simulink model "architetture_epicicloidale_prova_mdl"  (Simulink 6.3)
settings: Solver=ode45  StartTime=0.0  StopTime=3  RelTol=1e-3
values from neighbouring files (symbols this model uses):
  b_c = kb*J_c    (= 4.94590955184)    [architetture_epicicloidale.m]    (also in architetture_epicicloidale_cont.m; architetture_epicicloidale_HEV.m = 92.8974810391; architetture_epicicloidale_prova.m; architetture_HEV_controllo.m = 9.28974810391)
  b_r = kb*J_r    (= 218.026030555)    [architetture_epicicloidale.m]    (also in architetture_epicicloidale_cont.m; architetture_epicicloidale_HEV.m; architetture_epicicloidale_prova.m; architetture_HEV_controllo.m = 21.8026030555)
  b_s = kb*J_s    (= 8.12277148259)    [architetture_epicicloidale.m]    (also in architetture_epicicloidale_cont.m; architetture_epicicloidale_HEV.m = 4.94590955184; architetture_epicicloidale_prova.m; architetture_HEV_controllo.m = 0.494590955184)
  b_sc = kb*J_sc    (= 92.8974810391)    [architetture_epicicloidale.m]    (also in architetture_epicicloidale_cont.m; architetture_epicicloidale_prova.m; epicicloidale.m; epicicloidale_da_solo.m)
  bm = 0.8*N*metri*secondo/rad    (= 0.8)    [architetture_epicicloidale.m]    (also in architetture_epicicloidale_cont.m; architetture_epicicloidale_HEV.m; architetture_epicicloidale_prova.m; architetture_HEV_controllo.m)
  d_cs = d0    (= 10)    [architetture_epicicloidale.m]    (also in architetture_epicicloidale_cont.m; architetture_epicicloidale_prova.m; epicicloidale.m; epicicloidale_da_solo.m)
  d_sr = d0    (= 10)    [architetture_epicicloidale.m]    (also in architetture_epicicloidale_cont.m; architetture_epicicloidale_prova.m; epicicloidale.m; epicicloidale_da_solo.m)
  I_m = eye(m-1)    [architetture_epicicloidale.m]    (also in architetture_epicicloidale_cont.m; architetture_epicicloidale_HEV.m; architetture_epicicloidale_prova.m; architetture_HEV_controllo.m)
  Iw0 = 0*wI0    [architetture_epicicloidale.m]    (also in architetture_epicicloidale_cont.m = wI0; architetture_epicicloidale_HEV.m; architetture_epicicloidale_prova.m; architetture_HEV_controllo.m)
  J_c = 1.3*0.5*pi*rho_acc*hc*r_c^4    (= 0.0494590955184)    [architetture_epicicloidale.m]    (also in architetture_epicicloidale_cont.m; architetture_epicicloidale_HEV.m = 0.928974810391; architetture_epicicloidale_prova.m; architetture_HEV_controllo.m = 0.928974810391)
  J_r = 0.5*pi*rho_acc*(hr*r_ri^4 + h_ring*(r_re^4-r_ri^4))    (= 2.18026030555)    [architetture_epicicloidale.m]    (also in architetture_epicicloidale_cont.m; architetture_epicicloidale_HEV.m; architetture_epicicloidale_prova.m; architetture_HEV_controllo.m)
  J_s = Nr_sat*0.5*pi*rho_acc*(hs*r_s^4 + hc*r_s^4)    (= 0.0812277148259)    [architetture_epicicloidale.m]    (also in architetture_epicicloidale_cont.m; architetture_epicicloidale_HEV.m = 0.0494590955184; architetture_epicicloidale_prova.m; architetture_HEV_controllo.m = 0.0494590955184)
  J_sc = Nr_sat*(r_c+r_s)^2*rho_acc*pi*(hs*r_s^2 + hc*r_s^2)    (= 0.928974810391)    [architetture_epicicloidale.m]    (also in architetture_epicicloidale_cont.m; architetture_epicicloidale_prova.m; epicicloidale.m; epicicloidale_da_solo.m)
  Jm = 1.6*kg*metri^2    (= 1.6)    [architetture_epicicloidale.m]    (also in architetture_epicicloidale_cont.m; architetture_epicicloidale_HEV.m = 1.64945909552; architetture_epicicloidale_prova.m; architetture_HEV_controllo.m = 0.529459095518)
  Jr = Jr([1:m-1],[1:m-1])    [architetture_epicicloidale.m]    (also in architetture_epicicloidale_cont.m; architetture_epicicloidale_HEV.m; architetture_epicicloidale_prova.m; architetture_HEV_controllo.m)
  K_cs = K0    (= 10000000)    [architetture_epicicloidale.m]    (also in architetture_epicicloidale_cont.m; architetture_epicicloidale_prova.m; epicicloidale.m; epicicloidale_da_solo.m)
  K_sr = K0    (= 10000000)    [architetture_epicicloidale.m]    (also in architetture_epicicloidale_cont.m; architetture_epicicloidale_prova.m; epicicloidale.m; epicicloidale_da_solo.m)
  Kf = diag(diag(MLb)'./fliplr(tau_m(1:m-1)))    [architetture_epicicloidale_cont.m]    (also in architetture_epicicloidale_HEV.m; architetture_epicicloidale_prova.m; architetture_HEV_controllo.m; architetture_HEV_startstop.m)
  Kr = Kr([1:m-1])    [architetture_epicicloidale.m]    (also in architetture_epicicloidale_cont.m; architetture_epicicloidale_HEV.m; architetture_epicicloidale_prova.m; architetture_HEV_controllo.m)
  Li = 0.1*Henry    (= 0.1)    [architetture_epicicloidale.m]    (also in architetture_epicicloidale_cont.m; architetture_epicicloidale_HEV.m; architetture_epicicloidale_prova.m; architetture_HEV_controllo.m)
  m = 5    [architetture_epicicloidale.m]    (also in architetture_epicicloidale_cont.m; architetture_epicicloidale_HEV.m; architetture_epicicloidale_prova.m; architetture_HEV_controllo.m)
  Mi = 0.08*Henry    (= 0.08)    [architetture_epicicloidale.m]    (also in architetture_epicicloidale_cont.m; architetture_epicicloidale_HEV.m; architetture_epicicloidale_prova.m; architetture_HEV_controllo.m)
  MKr = MKr([1:m-1],[1:m-1])    [architetture_epicicloidale.m]    (also in architetture_epicicloidale_cont.m; architetture_epicicloidale_HEV.m; architetture_epicicloidale_prova.m; architetture_HEV_controllo.m)
  MLb = MLb([1:m-1],[1:m-1])    [architetture_epicicloidale.m]    (also in architetture_epicicloidale_cont.m; architetture_epicicloidale_HEV.m; architetture_epicicloidale_prova.m; architetture_HEV_controllo.m)
  MR = MR([1:m-1],[1:m-1])    [architetture_epicicloidale.m]    (also in architetture_epicicloidale_cont.m; architetture_epicicloidale_HEV.m; architetture_epicicloidale_prova.m; architetture_HEV_controllo.m)
  Nar = 200    [architetture_epicicloidale.m]    (also in architetture_epicicloidale_cont.m; architetture_epicicloidale_HEV.m; architetture_epicicloidale_prova.m; architetture_HEV_controllo.m)
  Nc = 30    [architetture_epicicloidale.m]    (also in architetture_epicicloidale_cont.m; architetture_epicicloidale_HEV.m; architetture_epicicloidale_prova.m; architetture_HEV_controllo.m)
  Nr_sat = 4    [architetture_epicicloidale.m]    (also in architetture_epicicloidale_cont.m; architetture_epicicloidale_HEV.m; architetture_epicicloidale_prova.m; architetture_HEV_controllo.m)
  p = 1    [architetture_epicicloidale.m]    (also in architetture_epicicloidale_cont.m; architetture_epicicloidale_HEV.m; architetture_epicicloidale_prova.m; architetture_HEV_controllo.m)
  Phir = 0.02*Weber    (= 0.02)    [architetture_epicicloidale.m]    (also in architetture_epicicloidale_cont.m; architetture_epicicloidale_HEV.m; architetture_epicicloidale_prova.m; architetture_HEV_controllo.m)
  r_c = r_ri-2*r_s    (= 0.101859163579)    [architetture_epicicloidale.m]    (also in architetture_epicicloidale_cont.m; architetture_epicicloidale_prova.m; epicicloidale.m; epicicloidale_da_solo.m)
  r_ri = xds*Nr/(2*pi)    (= 0.248281711223)    [architetture_epicicloidale.m]    (also in architetture_epicicloidale_cont.m; architetture_epicicloidale_prova.m; epicicloidale.m; epicicloidale_da_solo.m)
  r_s = xds*Ns/(2*pi)    (= 0.0732112738223)    [architetture_epicicloidale.m]    (also in architetture_epicicloidale_cont.m; architetture_epicicloidale_HEV.m = 0.101859163579; architetture_epicicloidale_prova.m; architetture_HEV_controllo.m = 0.101859163579)
  Ri = 3*Ohm    (= 3)    [architetture_epicicloidale.m]    (also in architetture_epicicloidale_cont.m; architetture_epicicloidale_HEV.m; architetture_epicicloidale_prova.m; architetture_HEV_controllo.m = 0.1)
  Star = Si    [architetture_epicicloidale.m]    (also in architetture_epicicloidale_cont.m; architetture_epicicloidale_HEV.m; architetture_epicicloidale_prova.m; architetture_HEV_controllo.m)
  Tau_sc = 200*N*metri    (= 200)    [architetture_epicicloidale.m]    (also in architetture_epicicloidale_cont.m = 50; architetture_epicicloidale_prova.m = 50; epicicloidale.m = 4; epicicloidale_da_solo.m = 4)
  Tc = 0.05*ms    (= 5e-05)    [architetture_epicicloidale.m]    (also in architetture_epicicloidale_cont.m; architetture_epicicloidale_HEV.m; architetture_epicicloidale_prova.m; architetture_HEV_controllo.m)
  Thm0 = 0    [architetture_epicicloidale.m]    (also in architetture_epicicloidale_cont.m; architetture_epicicloidale_HEV.m; architetture_epicicloidale_prova.m; architetture_HEV_controllo.m)
  tTb = tTb(:,[1:m-1])    [architetture_epicicloidale.m]    (also in architetture_epicicloidale_cont.m; architetture_epicicloidale_HEV.m; architetture_epicicloidale_prova.m; architetture_HEV_controllo.m)
  Wc_0 = 0*0.1*rad/secondo    (= 0)    [architetture_epicicloidale.m]    (also in architetture_epicicloidale_cont.m; architetture_epicicloidale_HEV.m; architetture_epicicloidale_prova.m; Confronto_CVT_EMR.m)
  Wm0 = 0*Wr_d    (= 0)    [architetture_epicicloidale.m]    (also in architetture_epicicloidale_cont.m = 62.5; architetture_epicicloidale_HEV.m; architetture_epicicloidale_prova.m; architetture_HEV_controllo.m)
  Wr_0 = Sys1.C(3,:)*[Wc_0; Wsc_0]    [architetture_epicicloidale.m]    (also in Confronto_CVT_EMR.m = 0; epicicloidale.m; epicicloidale_confronto_statico_elastico.m = [-r_s/r_r, 1+r_s/r_r]*[Ws_0; Wc_0]; epicicloidale_da_solo.m = [ -1/r_ri*r_c, (r_c+r_ri)/r_ri]*[Wc_0; Wsc_0])
  Wsc_0 = -0*0.2*rad/secondo    (= 0)    [architetture_epicicloidale.m]    (also in architetture_epicicloidale_cont.m; architetture_epicicloidale_HEV.m; architetture_epicicloidale_prova.m; epicicloidale.m = -0.2)
undefined symbols (not defined in the file or in its folder): a_0, a_1, B_Pneumatico, DFKc_max, eps_sk, K_Pneumatico, Lambda_mu, Mass_Matrix, Massa_Corpo_Auto, Mu_lambda, Raggio_Ruota_Ant, Raggio_Ruota_Pos, T_omega, tau_a0
libraries: simulink x11, dspmtrx3 x4, Tire_Soil x2, POG_Sincronous_Motors x1

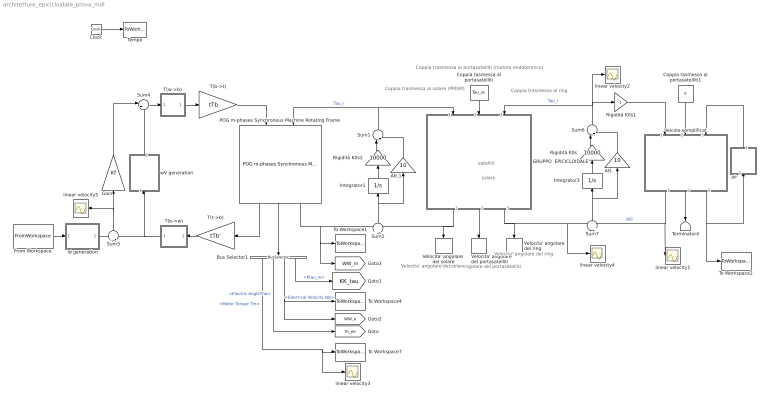
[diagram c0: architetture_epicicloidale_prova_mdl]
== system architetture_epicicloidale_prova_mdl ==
  note: solare
  note: satelliti
  note: Velocita' angolare del portasatelliti
  note: Velocita' angolare del ring
  note: Velocita' angolare del solare
  note: Coppia trasmessa al ring
  note: Coppia trasmessa al solare (PMSM)
  note: Coppia trasmessa ai portasatelliti (motore endotermico)
  " Id generation" : Subsystem
  Att. : Gain  Orientation=up  Gain=10
  Att.1 : Gain  Orientation=up  Gain=10
  Bus Selector1 : BusSelector  Orientation=down  OutputSignals=Motor Torque Tm,Electric AngleThe,Electrical Velocity We,Ktau_w
  Clock : Clock
  Coppia tasmessa al portasatelliti : Constant  Orientation=down  Value=Tau_sc
  Coppia tasmessa al portasatelliti1 : Constant  Orientation=down  Value=0
  From Workspace : FromWorkspace  VariableName=[T_in Tau_des]  SampleTime=0
  GRUPPO  EPICICLOIDALE : Subsystem  Orientation=down  mask(POG Gruppo epicicloidale){Par_solare=[J_c, b_c, r_c], Par_satelliti=[J_s, J_sc, b_s, b_sc, r_s, Nr_sat], Par_ring=[J_r, b_r, r_ri], Tipo_di_Modello=Modello ridotto Wc-Wsc, Cond_in_Wc_Wsc=[Wc_0,  Wsc_0], Cond_in_Wsc_Wr=[Wsc_0,  Wr_0], Cond_in_Wc_Wr=[Wc_0,  Wr_0], Solare_Satelliti=[K_cs, d_cs], Satelliti_Ring=[K_sr, d_sr], Cond_in=[Wc_0, Wsc_0,Wr_0]}
      mask prompts: Par_solare "Parametri Solare: [J_c, b_c, r_c]-->[kg*m^2,N*m*s/rad,m]"; Par_satelliti "Parametri Satelliti: [J_s, J_sc, b_s, b_sc, r_s, Nr_sat]-->[kg*m^2,N*m*s/rad,m]"; Par_ring "Parametri Ring: [J_r, b_r, r_ri]-->[kg*m^2,N*m*s/rad,m,m]"; Tipo_di_Modello "Tipo di modello"; Cond_in_Wc_Wsc "Condizioni iniziali: [Wc_0,  Wsc_0]-->[rad/s]"; Cond_in_Wsc_Wr "Condizioni iniziali: [Wsc_0,  Wr_0]-->[rad/s]"; Cond_in_Wc_Wr "Condizioni iniziali: [Wc_0,  Wr_0]-->[rad/s]"; Solare_Satelliti "Solare-Satelliti: [K_cs, d_cs]-->[N/m,N*m*s/rad]"; Satelliti_Ring "Satelliti-Ring: [K_sr, d_sr]-->[N/m,N*m*s/rad]"; Cond_in "Condizioni iniziali: [Wc_0,  Wsc_0, Wr_0]-->[rad/s]"
      mask help: Gruppo epicicloidale: [J_c, J_s, J_r, J_sc]= Inerzie di: solare, satelliti, ring, solare-ssatelliti; [b_c, b_s, b_r]= Attriti di: solare, satelliti, ring; [r_c, r_s, r_ri, r_re]= Raggi di: solare, satelliti, ring(interno ed esterno); [Nr_sat]= Numero Satelliti; [K_cs, K_sr]= Elasticita' tra solare-satelliti e tra satelliti-ring; [b_sc]= Attriti tra solare-satelliti; [d_cs, d_sr]= Elementi della matrice D; [Wc_0, Wsc_0, Wr_0]=Velocita' iniziali di solare, satelliti, portasatelliti, ring;
      mask init:
      | J_c=double(Par_solare(1));          
      | b_c=double(Par_solare(2));            
      | r_c=double(Par_solare(3));           
      | %
      | J_s=double(Par_satelliti(1));            
      | J_sc=double(Par_satelliti(2));            
      | b_s=double(Par_satelliti(3));            
      | b_sc=double(Par_satelliti(4));            
      | r_s=double(Par_satelliti(5));            
      | Nr_sat=double(Par_satelliti(6));           
      | %
      | J_r=double(Par_ring(1));             
      | b_r=double(Par_ring(2));            
      | r_ri=double(Par_ring(3));                  
      | %
      | %%%%%%%%%%%%%%%%%%%%%%%%%%%%%%%%%%%%%%%%%%%%%%%%%%%%%%%%%%%%%%%%%%%%%%%%%%%
      | %   Modello esteso e modelli ridotti
      | %%%%%%%%%%%%%%%%%%%%%%%%%%%%%%%%%%%%%%%%%%%%%%%%%%%%%%%%%%%%%%%%%%%%%%%%%%%
      | if Tipo_di_Modello=='Modello esteso        '
      |     %
      |     K_cs=double(Solare_Satelliti(1));
      |     d_cs=double(Solare_Satelliti(2));
      |     if(K_cs==0)
      |         K_cs=inf;
      |     end
      |     %
      |     K_sr=double(Satelliti_Ring(1));
      |     d_sr=double(Satelliti_Ring(2));
      |     if(K_sr==0)
      |         K_sr=inf;
      |     end
      |     %
      |     %
      |     L=[ J_c,      0,      0,      0,      0,      0;
      |           0, 1/K_cs,      0,      0,      0,      0;
      |           0,      0,    J_s,      0,      0,      0;
      |           0,      0,      0,   J_sc,      0,      0;
      |           0,      0,      0,      0, 1/K_sr,      0;
      |           0,      0,      0,      0,      0,    J_r];
      |     %
      |     A=- [-b_c-r_c^2*d_cs,    -r_c,                -r_c*d_cs*r_s,                   r_c^2*d_cs,      0,                  0;
      |         r_c,                    0,                          r_s,                         -r_c,      0,                  0;
      |         -r_c*d_cs*r_s,       -r_s,   -b_s-d_cs*r_s^2-d_sr*r_s^2,   r_c*d_cs*r_s-d_sr*r_s*r_ri,   -r_s,      d_sr*r_s*r_ri;
      |         r_c^2*d_cs,           r_c,   r_c*d_cs*r_s-d_sr*r_s*r_ri, -b_sc-r_c^2*d_cs-d_sr*r_ri^2,  -r_ri,        d_sr*r_ri^2;
      |         0,                      0,                          r_s,                         r_ri,      0,              -r_ri;
      |         0,                      0,                d_sr*r_s*r_ri,                  d_sr*r_ri^2,   r_ri,   -b_r-d_sr*r_ri^2];
      |     %
      |     B=[ 1, 0, 0;
      |         0, 0, 0;
      |         0, 0, 0;
      |         0, 1, 0;
      |         0, 0, 0;
      |         0, 0, 1];
      |     %
      |     C=[ 1, 0, 0, 0, 0, 0;
      |         0, 0, 0, 1, 0, 0;
      |         0, 0, 0, 0, 0, 1];
      |     %
      |     Wc_0=double(Cond_in(1));
      |     Wsc_0=double(Cond_in(2));
      |     Wr_0=double(Cond_in(3));
      |     Ws_0=r_c*(Wsc_0-Wc_0)/r_s;
      |     Ws_sc_0=[Ws_0 Wsc_0];
      |     %
      |     We_0=[Wc_0 0 Ws_sc_0 0 Wr_0 ];
      |     %
      | elseif Tipo_di_Modello=='Modello ridotto Wc-Wsc'
      |     L = [ (J_c*r_s^2*r_ri^2+r_ri^2*r_c^2*J_s+J_r*r_s^2*r_c^2)/r_s^2/r_ri^2,                                        -r_c*(r_ri^2*r_c*J_s+J_r*r_s^2*r_c+J_r*r_s^2*r_ri)/r_s^2/r_ri^2;
      |           -r_c*(r_ri^2*r_c*J_s+J_r*r_s^2*r_c+J_r*r_s^2*r_ri)/r_s^2/r_ri^2, (J_r*r_s^2*r_c^2+2*J_r*r_s^2*r_ri*r_c+J_r*r_s^2*r_ri^2+r_ri^2*r_c^2*J_s+r_ri^2*J_sc*r_s^2)/r_s^2/r_ri^2];
      |     %
      |     A=-[ -(b_c*r_s^2*r_ri^2+r_c^2*r_ri^2*b_s+b_r*r_s^2*r_c^2)/r_s^2/r_ri^2,                                          r_c*(r_c*r_ri^2*b_s+b_r*r_s^2*r_c+b_r*r_s^2*r_ri)/r_s^2/r_ri^2;
      |         r_c*(r_c*r_ri^2*b_s+b_r*r_s^2*r_c+b_r*r_s^2*r_ri)/r_s^2/r_ri^2,    -(b_sc*r_s^2*r_ri^2+r_c^2*r_ri^2*b_s+b_r*r_s^2*r_c^2+2*b_r*r_s^2*r_c*r_ri+b_r*r_s^2*r_ri^2)/r_s^2/r_ri^2];
      |     %
      |     B= [  1,    0,     -1/r_ri*r_c;
      |           0,    1, (r_c+r_ri)/r_ri];
      |     %
      |     C= [            1,               0;
      |                     0,               1;
      |           -1/r_ri*r_c, (r_c+r_ri)/r_ri];
      |     %
      |     Wc_0=double(Cond_in_Wc_Wsc(1));
      |     Wsc_0=double(Cond_in_Wc_Wsc(2));
      |     We_0=[Wc_0 Wsc_0];
      |     %
      | elseif Tipo_di_Modello=='Modello ridotto Wsc-Wr'
      |     L= [ (J_sc*r_c^2*r_s^2+J_c*r_s^2*r_c^2+2*J_c*r_s^2*r_c*r_ri+J_c*r_s^2*r_ri^2+r_ri^2*J_s*r_c^2)/r_c^2/r_s^2,   -r_ri*(J_c*r_s^2*r_c+J_c*r_s^2*r_ri+r_ri*J_s*r_c^2)/r_c^2/r_s^2;
      |          -r_ri*(J_c*r_s^2*r_c+J_c*r_s^2*r_ri+r_ri*J_s*r_c^2)/r_c^2/r_s^2,                                        (J_r*r_c^2*r_s^2+J_c*r_s^2*r_ri^2+r_ri^2*J_s*r_c^2)/r_c^2/r_s^2];
      | 
      |     A=-[ -(b_sc*r_c^2*r_s^2+b_c*r_s^2*r_c^2+2*b_c*r_s^2*r_c*r_ri+b_c*r_s^2*r_ri^2+r_ri^2*b_s*r_c^2)/r_c^2/r_s^2,     r_ri*(b_c*r_s^2*r_c+b_c*r_s^2*r_ri+r_ri*b_s*r_c^2)/r_c^2/r_s^2;
      |          r_ri*(b_c*r_s^2*r_c+b_c*r_s^2*r_ri+r_ri*b_s*r_c^2)/r_c^2/r_s^2,                                          -(b_r*r_c^2*r_s^2+b_c*r_s^2*r_ri^2+r_ri^2*b_s*r_c^2)/r_c^2/r_s^2];
      | 
      |     B= [ (r_c+r_ri)/r_c,    1,   0;
      |             -1/r_c*r_ri,    0,   1];
      | 
      |     C= [ (r_c+r_ri)/r_c,  -1/r_c*r_ri;
      |                       1,            0;
      |                       0,            1];
      |     %
      |     Wsc_0=double(Cond_in_Wsc_Wr(1));
      |     Wr_0=double(Cond_in_Wsc_Wr(2));
      |     We_0=[Wsc_0 Wr_0];
      |     %
      | elseif Tipo_di_Modello=='Modello ridotto  Wc-Wr'
      |     L= [ (J_c*r_s^2*r_c^2+2*J_c*r_s^2*r_c*r_ri+J_c*r_s^2*r_ri^2+r_ri^2*r_c^2*J_s+r_c^2*J_sc*r_s^2)/r_s^2/(r_c+r_ri)^2,                                                        r_c*r_ri*(-r_ri*r_c*J_s+J_sc*r_s^2)/r_s^2/(r_c+r_ri)^2;
      |           r_c*r_ri*(-r_ri*r_c*J_s+J_sc*r_s^2)/r_s^2/(r_c+r_ri)^2,                                                      (J_r*r_s^2*r_c^2+2*J_r*r_s^2*r_c*r_ri+J_r*r_s^2*r_ri^2+r_ri^2*r_c^2*J_s+r_ri^2*J_sc*r_s^2)/r_s^2/(r_c+r_ri)^2];
      | 
      |     A=-[-(b_c*r_s^2*r_c^2+2*b_c*r_s^2*r_c*r_ri+b_c*r_s^2*r_ri^2+r_c^2*r_ri^2*b_s+r_c^2*r_s^2*b_sc)/r_s^2/(r_c+r_ri)^2,                                                        -r_c*r_ri*(-r_c*r_ri*b_s+r_s^2*b_sc)/r_s^2/(r_c+r_ri)^2;
      |         -r_c*r_ri*(-r_c*r_ri*b_s+r_s^2*b_sc)/r_s^2/(r_c+r_ri)^2,                                                       -(b_r*r_s^2*r_c^2+2*b_r*r_s^2*r_c*r_ri+b_r*r_s^2*r_ri^2+r_c^2*r_ri^2*b_s+r_ri^2*r_s^2*b_sc)/r_s^2/(r_c+r_ri)^2];
      | 
      |     B=[   1,  1/(r_c+r_ri)*r_c, 0;
      |           0, 1/(r_c+r_ri)*r_ri, 1];
      | 
      |     C=[                 1,                  0;
      |          1/(r_c+r_ri)*r_c,  1/(r_c+r_ri)*r_ri;
      |                         0,                  1];
      |     Wc_0=double(Cond_in_Wc_Wr(1));
      |     Wr_0=double(Cond_in_Wc_Wr(2));
      |     We_0=[Wc_0 Wr_0];
      | end
  Gain : Gain  Orientation=up  Gain=Kf  Multiplication=Matrix(K*u) (u vector)
  Integrator1 : Integrator  Orientation=up
  Integrator3 : Integrator  Orientation=up
  POG m-phases Synchronous Machine Rotating Frame : POG_Sincronous_Motors/POG m-phases Synchronous Machine Rotating Frame  Orientation=down  Motor_Par=[m p]  Phase_Par=[Nc Star]  Electric_Par=[Ri Li Mi]  Mech_Par=[Jm bm]  Plux_Par=[Phir Nar]  Iniz_Cond=[Wm0; Thm0; Iw0]  TipoFlux=User defined  Tipo=Tipo  alfa=al  degree=6  TipoF=Tipo
  Rigidità K0s : Gain  Orientation=up  Gain=10000
  Rigidità K0s1 : Gain  Gain=-1
  Rigidità K0s2 : Gain  Orientation=up  Gain=10000
  Sum1 : Sum  Orientation=up  Inputs=|++
  Sum2 : Sum  Orientation=up  Inputs=+|-
  Sum3 : Sum  Orientation=up  Inputs=+|-
  Sum4 : Sum  Inputs=|++
  Sum6 : Sum  Orientation=up  Inputs=|++
  Sum7 : Sum  Orientation=up  Inputs=-|+
  T(b->t) : Gain  Gain=tTb  Multiplication=Matrix(K*u) (u vector)
  T(b->w) : Subsystem  Orientation=left  AncestorBlock=|
      | POG_Electric_Bloks/POG m-phases
      | Synchronous Machine
      | Rotating Frame/T(b->w)
  T(t->b) : Gain  Orientation=left  Gain=tTb'  Multiplication=Matrix(K*u) (u vector)
  T(w->b) : Subsystem  AncestorBlock=|
      | POG_Electric_Bloks/POG m-phases
      | Synchronous Machine
      | Rotating Frame/T(w->b)
  Tempo : ToWorkspace  VariableName=t  SampleTime=Tc  SaveFormat=Array
  Terminator4 : Terminator
  To Workspace1 : ToWorkspace  VariableName=Wm  SampleTime=Tc  SaveFormat=Array
  To Workspace2 : ToWorkspace  VariableName=Vvehicle  SampleTime=Tc  SaveFormat=Array
  To Workspace4 : ToWorkspace  VariableName=We  SampleTime=Tc  SaveFormat=Array
  To Workspace7 : ToWorkspace  VariableName=Tm  SampleTime=Tc  SaveFormat=Array
  Veicolo semplificat : Subsystem  Orientation=down
  Velocita' angolare del ring : ToWorkspace  VariableName=W_r  SampleTime=Tc  SaveFormat=Array
  Velocita' angolare  del portasatelliti : ToWorkspace  VariableName=W_sc  SampleTime=Tc  SaveFormat=Array
  Velocita' angolare  del solare : ToWorkspace  VariableName=W_c  SampleTime=Tc  SaveFormat=Array
  air : Subsystem  Orientation=up
  linear velocity{1..5} (5 alike) : Scope
  wV generation : Subsystem  Orientation=up
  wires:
  Clock/1 -> Tempo/1
  Coppia tasmessa al portasatelliti/1 -> GRUPPO  EPICICLOIDALE/2(Tau_sc)
  GRUPPO  EPICICLOIDALE/3(w_r) -> Velocita' angolare del ring/1, Sum7/1, linear velocity4/1
  GRUPPO  EPICICLOIDALE/2(w_sc) -> Velocita' angolare  del portasatelliti/1
  GRUPPO  EPICICLOIDALE/1(w_c) -> Velocita' angolare  del solare/1, Sum2/2
  POG m-phases Synchronous Machine Rotating Frame/3 -> Sum2/1, To Workspace1/1, [WW_m]
  POG m-phases Synchronous Machine Rotating Frame/2 -> Bus Selector1/1
  Bus Selector1/3 -> To Workspace4/1, [WW_e]  "<Electrical Velocity We>"
  T(w->b)/1(It) -> T(b->t)/1
  T(b->t)/1 -> POG m-phases Synchronous Machine Rotating Frame/1
  T(t->b)/1 -> T(b->w)/1(Vt)
  T(b->w)/1(Vw) -> wV generation/1(In1), Sum3/2
  POG m-phases Synchronous Machine Rotating Frame/1 -> T(t->b)/1
  Bus Selector1/2 -> [th_ee]  "<Electric AngleThe>"
  Bus Selector1/1 -> To Workspace7/1, linear velocity3/1  "<Motor Torque Tm>"
  Att./1 -> Sum6/2
  Rigidità K0s/1 -> Sum6/1
  Integrator3/1 -> Rigidità K0s/1
  Sum6/1 -> linear velocity2/1, Rigidità K0s1/1, GRUPPO  EPICICLOIDALE/3(Tau_r)  "Tau_r"
  Sum7/1 -> Att./1, Integrator3/1
  Coppia tasmessa al portasatelliti1/1 -> Veicolo semplificat/2(Tau2)
  Rigidità K0s1/1 -> Veicolo semplificat/1(Tau1)
  Att.1/1 -> Sum1/2
  Rigidità K0s2/1 -> Sum1/1
  Integrator1/1 -> Rigidità K0s2/1
  Sum2/1 -> Att.1/1, Integrator1/1
  Sum1/1 -> POG m-phases Synchronous Machine Rotating Frame/2, GRUPPO  EPICICLOIDALE/1(Tau_c)  "Tau_r"
  " Id generation"/1(Out1) -> Sum3/1
  Sum3/1 -> Gain/1, linear velocity5/1
  Sum4/1 -> T(w->b)/1(Iw)
  From Workspace/1 -> " Id generation"/1(In1)
  Gain/1 -> Sum4/1
  wV generation/1(Out1) -> Sum4/2
  Veicolo semplificat/1(W1) -> Sum7/2, linear velocity1/1  "W0"
  Veicolo semplificat/3(V) -> To Workspace2/1, air/1(In1)
  Bus Selector1/4 -> [KK_tau]  "<Ktau_w>"
  air/1(Out1) -> Veicolo semplificat/3(Fres)
  Veicolo semplificat/2(W2) -> Terminator4/1

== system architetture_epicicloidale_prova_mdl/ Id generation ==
  In1 : Inport
  Divide : Product  Inputs=*/  OutScaling=2^-10
  Product : Product
  modulo : Subsystem
  versore : Subsystem
  Out1 : Outport
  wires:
  [KK_tau] -> modulo/1(In1), versore/1(In1)
  modulo/1(Out1) -> Divide/2
  Divide/1 -> Product/1
  versore/1(Out1) -> Product/2
  In1/1 -> Divide/1
  Product/1 -> Out1/1

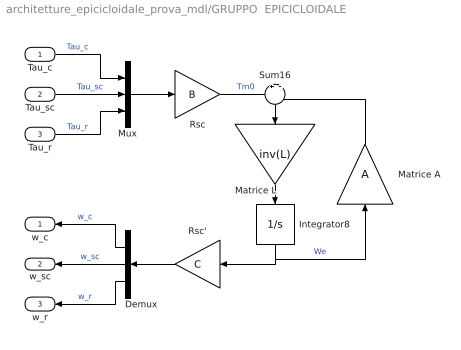
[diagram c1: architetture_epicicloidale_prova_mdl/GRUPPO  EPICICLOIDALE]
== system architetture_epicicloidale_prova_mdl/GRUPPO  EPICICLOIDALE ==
  Tau_c : Inport
  Tau_sc : Inport  Port=2
  Tau_r : Inport  Port=3
  Demux : Demux  Orientation=left  Outputs=3
  Integrator8 : Integrator  Orientation=down  InitialCondition=We_0  LowerSaturationLimit=0
  Matrice A : Gain  Orientation=up  Gain=A  Multiplication=Matrix(K*u)
  Matrice L : Gain  Orientation=down  Gain=inv(L)  Multiplication=Matrix(K*u)
  Mux : Mux  Inputs=3
  Rsc : Gain  Gain=B  Multiplication=Matrix(K*u)
  Rsc' : Gain  Orientation=left  Gain=C  Multiplication=Matrix(K*u)
  Sum16 : Sum  Orientation=down  Inputs=+|-
  w_c : Outport  Orientation=left
  w_sc : Outport  Orientation=left  Port=2
  w_r : Outport  Orientation=left  Port=3
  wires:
  Rsc/1 -> Sum16/1  "Tm0"
  Sum16/1 -> Matrice L/1
  Matrice L/1 -> Integrator8/1
  Integrator8/1 -> Matrice A/1, Rsc'/1  "We"
  Matrice A/1 -> Sum16/2
  Tau_c/1 -> Mux/1  "Tau_c"
  Tau_sc/1 -> Mux/2  "Tau_sc"
  Tau_r/1 -> Mux/3  "Tau_r"
  Mux/1 -> Rsc/1
  Rsc'/1 -> Demux/1
  Demux/1 -> w_c/1  "w_c"
  Demux/2 -> w_sc/1  "w_sc"
  Demux/3 -> w_r/1  "w_r"

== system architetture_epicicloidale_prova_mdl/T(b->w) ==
  Vt : Inport
  Product : Product  Multiplication=Matrix(*)
  Vw : Outport
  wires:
  Vt/1 -> Product/2
  Product/1 -> Vw/1
  [T_w_be] -> Product/1

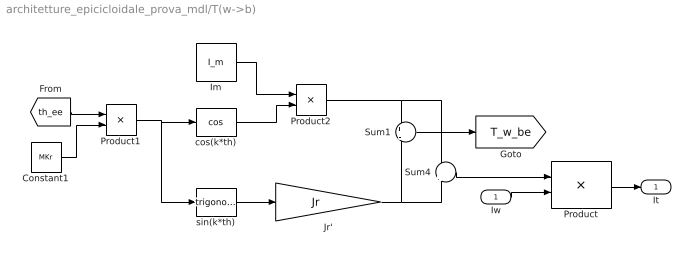
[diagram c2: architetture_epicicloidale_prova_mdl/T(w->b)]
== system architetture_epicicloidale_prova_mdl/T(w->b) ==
  Iw : Inport
  Constant1 : Constant  Value=MKr
  Im : Constant  Value=I_m  VectorParams1D=off
  Jr' : Gain  Gain=Jr  Multiplication=Matrix(K*u)
  Product : Product  Multiplication=Matrix(*)
  Product1 : Product
  Product2 : Product
  Sum1 : Sum  Inputs=+|-
  Sum4 : Sum  Inputs=+|+
  cos(k*th) : Trigonometry  Operator=cos
  sin(k*th) : Trigonometry
  It : Outport
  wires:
  Sum4/1 -> Product/1
  Product/1 -> It/1
  Iw/1 -> Product/2
  Jr'/1 -> Sum4/2, Sum1/2
  Product2/1 -> Sum4/1, Sum1/1
  Im/1 -> Product2/1
  cos(k*th)/1 -> Product2/2
  Product1/1 -> sin(k*th)/1, cos(k*th)/1
  Constant1/1 -> Product1/2
  [th_ee] -> Product1/1
  sin(k*th)/1 -> Jr'/1
  Sum1/1 -> [T_w_be]

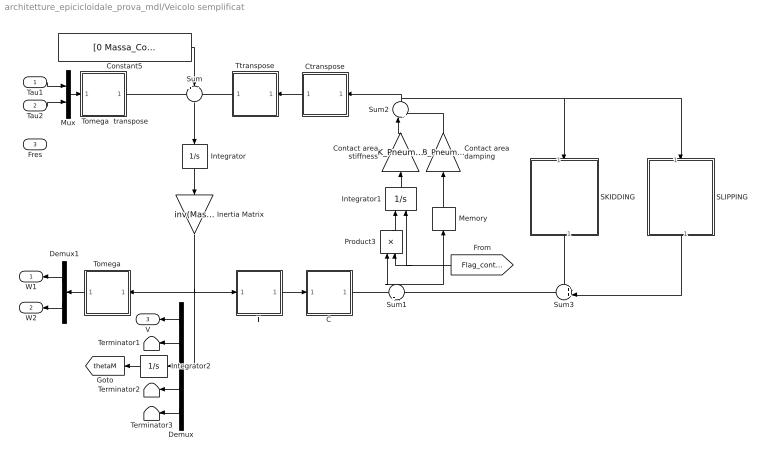
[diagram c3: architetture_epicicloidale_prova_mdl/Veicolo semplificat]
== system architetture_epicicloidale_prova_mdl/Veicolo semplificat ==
  Tau1 : Inport
  Tau2 : Inport  Port=2
  Fres : Inport  Port=3
  C : Subsystem
  Constant5 : Constant  Value=[0 Massa_Corpo_Auto*9.81 0 0 0]
  Contact area damping : Gain  Orientation=up  Gain=B_Pneumatico  Multiplication=Matrix(K*u) (u vector)
  Contact area stiffness : Gain  Orientation=up  Gain=K_Pneumatico  Multiplication=Matrix(K*u) (u vector)
  Ctranspose : Subsystem  Orientation=left
  Demux : Demux  Orientation=left  Outputs=5
  Demux1 : Demux  Orientation=left  Outputs=2
  Inertia Matrix : Gain  Orientation=down  Gain=inv(Mass_Matrix)  Multiplication=Matrix(K*u)
  Integrator : Integrator  Orientation=down  InitialCondition=[0 0 0 0 0]
  Integrator1 : Integrator  Orientation=up  ExternalReset=falling  InitialCondition=[0 0 0 0 0 0]
  Integrator2 : Integrator  Orientation=left
  Memory : Memory  Orientation=up
  Mux : Mux  Inputs=2
  Product3 : Product  Orientation=up  Inputs=**
  SKIDDING : Subsystem  Orientation=down  AncestorBlock=Tire_Soil/Tire-soil contact ENERGETIC/Contatto elastico/SKIDDING
  SLIPPING : Subsystem  Orientation=down  AncestorBlock=Tire_Soil/Tire-soil contact ENERGETIC/Contatto elastico/SLIPPING
  Sum : Sum  Orientation=down  Inputs=+--
  Sum1 : Sum  Orientation=up  Inputs=+-
  Sum2 : Sum  Orientation=up  Inputs=|++
  Sum3 : Sum  Orientation=left  Inputs=++|
  T : Subsystem
  Terminator1 : Terminator
  Terminator2 : Terminator
  Terminator3 : Terminator
  Tomega : Subsystem  Orientation=left
  Tomega  transpose : Subsystem
  Ttranspose : Subsystem  Orientation=left
  W1 : Outport  Orientation=left
  W2 : Outport  Orientation=left  Port=2
  V : Outport  Orientation=left  Port=3
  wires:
  Demux/5 -> Terminator3/1
  Demux/4 -> Terminator2/1
  Demux/2 -> Terminator1/1
  Demux/1 -> V/1
  Tomega/1(Vt) -> Demux1/1
  Tau2/1 -> Mux/2
  Tau1/1 -> Mux/1
  Mux/1 -> Tomega  transpose/1(T)
  Tomega  transpose/1(Tt) -> Sum/1
  Constant5/1 -> Sum/2
  Sum3/1 -> Sum1/2
  SKIDDING/1(Vcsk) -> Sum3/1
  SLIPPING/1(Vcsl) -> Sum3/2
  Memory/1 -> Contact area damping/1
  Integrator1/1 -> Contact area stiffness/1
  Product3/1 -> Integrator1/1
  [Flag_contatto] -> Integrator1/2, Product3/2
  C/1(Xcdot) -> Sum1/1
  Ctranspose/1(F) -> Ttranspose/1(F)
  T/1(Xdot) -> C/1(Xdot)
  Integrator2/1 -> [thetaM]
  Demux/3 -> Integrator2/1
  Contact area stiffness/1 -> Sum2/1
  Contact area damping/1 -> Sum2/2
  Sum1/1 -> Memory/1, Product3/1
  Sum2/1 -> Ctranspose/1(Fc), SLIPPING/1(Fxyz), SKIDDING/1(Fxyz)
  Ttranspose/1(Ft) -> Sum/3
  Inertia Matrix/1 -> T/1(V), Tomega/1(V), Demux/1
  Integrator/1 -> Inertia Matrix/1
  Sum/1 -> Integrator/1
  Demux1/1 -> W1/1
  Demux1/2 -> W2/1

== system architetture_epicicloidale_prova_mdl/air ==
  In1 : Inport  Orientation=up
  air : Fcn  Orientation=up  Expr=10*u^2
  Out1 : Outport  Orientation=up
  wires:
  In1/1 -> air/1
  air/1 -> Out1/1

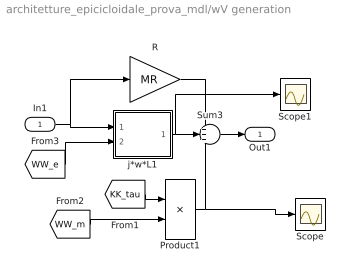
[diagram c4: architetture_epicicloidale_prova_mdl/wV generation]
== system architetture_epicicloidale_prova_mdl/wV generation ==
  In1 : Inport
  Product1 : Product  Multiplication=Matrix(*)
  R : Gain  Gain=MR  Multiplication=Matrix(K*u) (u vector)
  Scope : Scope
  Scope1 : Scope
  Sum3 : Sum  Inputs=+++
  j*w*L1 : Subsystem  AncestorBlock=|
      | POG_Electric_Bloks/POG m-phases
      | Synchronous Machine
      | Rotating Frame/j*w*L
  Out1 : Outport
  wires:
  [KK_tau] -> Product1/1
  [WW_m] -> Product1/2
  R/1 -> Sum3/1
  j*w*L1/1(Out1) -> Sum3/2, Scope1/1
  Product1/1 -> Sum3/3, Scope/1
  In1/1 -> j*w*L1/1(In1), R/1
  Sum3/1 -> Out1/1
  [WW_e] -> j*w*L1/2(In2)

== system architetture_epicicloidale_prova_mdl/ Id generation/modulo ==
  In1 : Inport
  Dot Product : simulink/Math Operations/Dot Product  InputSameDT=on  OutDataType=sfix(16)  OutScaling=2^-10  DoSatur=off
  Math Function : Math  Operator=sqrt
  Out1 : Outport
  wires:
  In1/1 -> Dot Product/1, Dot Product/2
  Dot Product/1 -> Math Function/1
  Math Function/1 -> Out1/1

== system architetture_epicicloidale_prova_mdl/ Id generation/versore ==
  In1 : Inport
  Constant : Constant  Value=0.0001
  Divide : Product  Inputs=*/  OutScaling=2^-10
  Norma  del vettore : Subsystem
  Sum1 : Sum  Inputs=|++
  Out1 : Outport
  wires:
  Divide/1 -> Out1/1  "versore"
  Constant/1 -> Sum1/2
  Sum1/1 -> Divide/2
  Norma  del vettore/1(Out1) -> Sum1/1
  In1/1 -> Norma  del vettore/1(In1), Divide/1

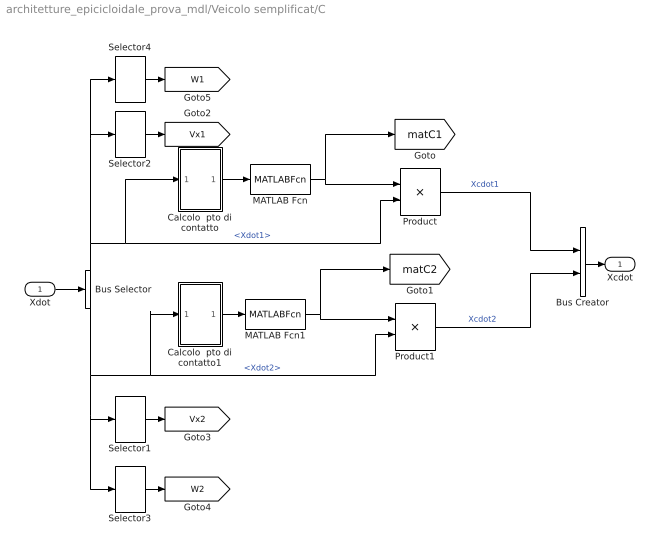
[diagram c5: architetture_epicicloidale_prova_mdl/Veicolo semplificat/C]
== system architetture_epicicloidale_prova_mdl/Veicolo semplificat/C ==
  Xdot : Inport
  Bus Creator : BusCreator  Inputs=2
  Bus Selector : BusSelector  OutputSignals=Xdot1,Xdot2
  Calcolo  pto di contatto : Subsystem
  Calcolo  pto di contatto1 : Subsystem
  MATLAB Fcn : MATLABFcn  MATLABFcn=matrice_c  Output1D=off
  MATLAB Fcn1 : MATLABFcn  MATLABFcn=matrice_c  Output1D=off
  Product : Product  Inputs=**  Multiplication=Matrix(*)
  Product1 : Product  Inputs=**  Multiplication=Matrix(*)
  Selector1 : Selector  InputPortWidth=3
  Selector2 : Selector  InputPortWidth=3
  Selector3 : Selector  Elements=3  InputPortWidth=3
  Selector4 : Selector  Elements=3  InputPortWidth=3
  Xcdot : Outport
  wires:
  Selector3/1 -> [W2]
  Selector4/1 -> [W1]
  Selector1/1 -> [Vx2]
  Selector2/1 -> [Vx1]
  Bus Creator/1 -> Xcdot/1
  Bus Selector/1 -> Selector4/1, Selector2/1, Product/2, Calcolo  pto di contatto/1(In1)  "<Xdot1>"
  Xdot/1 -> Bus Selector/1
  Calcolo  pto di contatto1/1(Out1) -> MATLAB Fcn1/1
  MATLAB Fcn1/1 -> [matC2], Product1/1
  Bus Selector/2 -> Selector3/1, Selector1/1, Calcolo  pto di contatto1/1(In1), Product1/2  "<Xdot2>"
  Product1/1 -> Bus Creator/2  "Xcdot2"
  Calcolo  pto di contatto/1(Out1) -> MATLAB Fcn/1
  MATLAB Fcn/1 -> [matC1], Product/1
  Product/1 -> Bus Creator/1  "Xcdot1"

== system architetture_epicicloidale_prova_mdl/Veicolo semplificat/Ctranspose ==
  Fc : Inport
  Mux : Mux  Inputs=2
  Product : Product  Inputs=**  Multiplication=Matrix(*)
  Product1 : Product  Inputs=**  Multiplication=Matrix(*)
  Selector : Selector  Elements=[1 2 3]  InputPortWidth=6
  Selector1 : Selector  Elements=[4 5 6]  InputPortWidth=6
  Transpose : dspmtrx3/Transpose  Hermitian=off  overflowFlag=on
  Transpose1 : dspmtrx3/Transpose  Hermitian=off  overflowFlag=on
  F : Outport
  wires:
  Selector1/1 -> Product1/2
  Selector/1 -> Product/2
  Fc/1 -> Selector1/1, Selector/1
  Mux/1 -> F/1
  Product1/1 -> Mux/2
  Product/1 -> Mux/1
  [matC2] -> Transpose1/1
  Transpose1/1 -> Product1/1
  [matC1] -> Transpose/1
  Transpose/1 -> Product/1

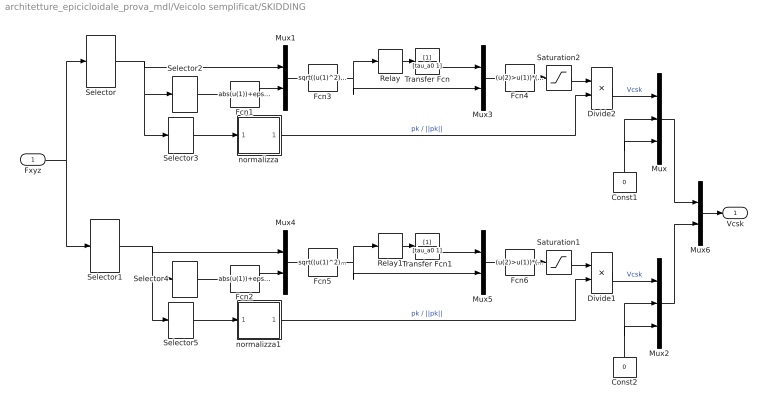
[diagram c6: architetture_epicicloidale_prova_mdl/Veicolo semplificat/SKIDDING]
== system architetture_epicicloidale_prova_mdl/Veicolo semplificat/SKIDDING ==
  Fxyz : Inport
  Const1 : Constant  Orientation=up  Value=0
  Const2 : Constant  Orientation=up  Value=0
  Divide1 : Product  Inputs=**  OutScaling=2^-10
  Divide2 : Product  Inputs=**  OutScaling=2^-10
  Fcn1 : Fcn  Expr=abs(u(1))+eps_sk
  Fcn2 : Fcn  Expr=abs(u(1))+eps_sk
  Fcn3 : Fcn  Expr=sqrt((u(1)^2))/u(4)
  Fcn4 : Fcn  Expr=(u(2)>u(1))*(u(2)-u(1))^2*Kc
  Fcn5 : Fcn  Expr=sqrt((u(1)^2))/u(4)
  Fcn6 : Fcn  Expr=(u(2)>u(1))*(u(2)-u(1))^2*Kc
  Mux : Mux  Inputs=3
  Mux{1,3..6} (5 alike) : Mux  Inputs=2
  Mux2 : Mux  Inputs=3
  Relay : Relay  OnSwitchValue=a_0  OffSwitchValue=a_1  OnOutputValue=a_1  OffOutputValue=a_0
  Relay1 : Relay  OnSwitchValue=a_0  OffSwitchValue=a_1  OnOutputValue=a_1  OffOutputValue=a_0
  Saturation1 : Saturate  UpperLimit=DFKc_max  LowerLimit=0
  Saturation2 : Saturate  UpperLimit=DFKc_max  LowerLimit=0
  Selector : Selector  Elements=[1 2 3]  InputPortWidth=6
  Selector1 : Selector  Elements=[4 5 6]  InputPortWidth=6
  Selector2 : Selector  Elements=[2]  InputPortWidth=3
  Selector3 : Selector  InputPortWidth=3
  Selector4 : Selector  Elements=[2]  InputPortWidth=3
  Selector5 : Selector  InputPortWidth=3
  Transfer Fcn : TransferFcn  Denominator=[tau_a0 1]
  Transfer Fcn1 : TransferFcn  Denominator=[tau_a0 1]
  normalizza : Subsystem
  normalizza1 : Subsystem
  Vcsk : Outport
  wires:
  Mux6/1 -> Vcsk/1
  Mux2/1 -> Mux6/2
  Mux/1 -> Mux6/1
  Const2/1 -> Mux2/3, Mux2/2
  Selector1/1 -> Mux4/1, Selector5/1, Selector4/1
  Divide1/1 -> Mux2/1  "Vcsk"
  Selector4/1 -> Fcn2/1
  Selector5/1 -> normalizza1/1(In1)
  normalizza1/1(Out1) -> Divide1/2  "pk / ||pk||"
  Saturation1/1 -> Divide1/1
  Fcn6/1 -> Saturation1/1
  Fcn5/1 -> Relay1/1, Mux5/2
  Mux4/1 -> Fcn5/1
  Fcn2/1 -> Mux4/2
  Mux5/1 -> Fcn6/1
  Relay1/1 -> Transfer Fcn1/1
  Transfer Fcn1/1 -> Mux5/1
  Const1/1 -> Mux/3, Mux/2
  Selector/1 -> Mux1/1, Selector3/1, Selector2/1
  Divide2/1 -> Mux/1  "Vcsk"
  Fxyz/1 -> Selector1/1, Selector/1
  Selector2/1 -> Fcn1/1
  Selector3/1 -> normalizza/1(In1)
  normalizza/1(Out1) -> Divide2/2  "pk / ||pk||"
  Saturation2/1 -> Divide2/1
  Fcn4/1 -> Saturation2/1
  Fcn3/1 -> Relay/1, Mux3/2
  Mux1/1 -> Fcn3/1
  Fcn1/1 -> Mux1/2
  Mux3/1 -> Fcn4/1
  Relay/1 -> Transfer Fcn/1
  Transfer Fcn/1 -> Mux3/1

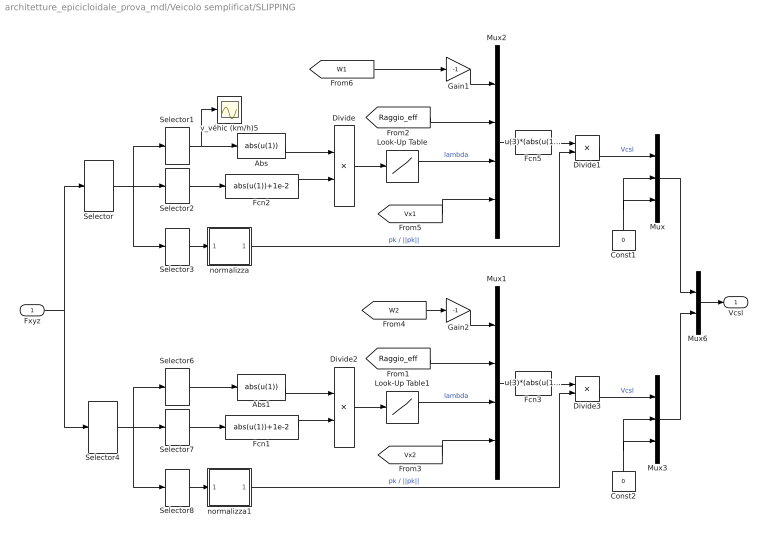
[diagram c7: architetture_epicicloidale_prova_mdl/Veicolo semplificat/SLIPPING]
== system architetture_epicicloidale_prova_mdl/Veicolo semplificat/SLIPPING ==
  Fxyz : Inport
  Abs : Fcn  Expr=abs(u(1))
  Abs1 : Fcn  Expr=abs(u(1))
  Const1 : Constant  Orientation=up  Value=0
  Const2 : Constant  Orientation=up  Value=0
  Divide : Product  Inputs=*/  OutScaling=2^-10
  Divide1 : Product  Inputs=**  OutScaling=2^-10
  Divide2 : Product  Inputs=*/  OutScaling=2^-10
  Divide3 : Product  Inputs=**  OutScaling=2^-10
  Fcn1 : Fcn  Expr=abs(u(1))+1e-2
  Fcn2 : Fcn  Expr=abs(u(1))+1e-2
  Fcn3 : Fcn  Expr=u(3)*(abs(u(1)*u(2))*(abs(u(1)*u(2))<=abs(u(4)))+abs(u(4))*(abs(u(1)*u(2))>abs(u(4))))
  Fcn5 : Fcn  Expr=u(3)*(abs(u(1)*u(2))*(abs(u(1)*u(2))<=abs(u(4)))+abs(u(4))*(abs(u(1)*u(2))>abs(u(4))))
  Gain1 : Gain  Gain=-1
  Gain2 : Gain  Gain=-1
  Look-Up Table : Lookup  InputValues=Mu_lambda  OutputValues=Lambda_mu
  Look-Up Table1 : Lookup  InputValues=Mu_lambda  OutputValues=Lambda_mu
  Mux : Mux  Inputs=3
  Mux1 : Mux
  Mux2 : Mux
  Mux3 : Mux  Inputs=3
  Mux6 : Mux  Inputs=2
  Selector : Selector  Elements=[1 2 3]  InputPortWidth=6
  Selector{1,3,6,8} (4 alike) : Selector  InputPortWidth=3
  Selector2 : Selector  Elements=[2]  InputPortWidth=3
  Selector4 : Selector  Elements=[4 5 6]  InputPortWidth=6
  Selector7 : Selector  Elements=[2]  InputPortWidth=3
  normalizza : Subsystem
  normalizza1 : Subsystem
  v_véhic (km/h)5 : Scope
  Vcsl : Outport
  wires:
  [W2] -> Gain2/1
  [W1] -> Gain1/1
  Mux6/1 -> Vcsl/1
  Mux3/1 -> Mux6/2
  Mux/1 -> Mux6/1
  Const2/1 -> Mux3/3, Mux3/2
  Divide3/1 -> Mux3/1  "Vcsl"
  Const1/1 -> Mux/2, Mux/3
  Divide1/1 -> Mux/1  "Vcsl"
  normalizza1/1(Out1) -> Divide3/2  "pk / ||pk||"
  Selector4/1 -> Selector6/1, Selector8/1, Selector7/1
  Selector7/1 -> Fcn1/1
  Selector8/1 -> normalizza1/1(In1)
  Fcn1/1 -> Divide2/2
  Abs1/1 -> Divide2/1
  Selector6/1 -> Abs1/1
  Look-Up Table1/1 -> Mux1/3  "lambda"
  Divide2/1 -> Look-Up Table1/1
  [Raggio_eff] -> Mux1/2
  Gain2/1 -> Mux1/1
  [Vx2] -> Mux1/4
  Mux1/1 -> Fcn3/1
  Fcn3/1 -> Divide3/1
  Fxyz/1 -> Selector4/1, Selector/1
  normalizza/1(Out1) -> Divide1/2  "pk / ||pk||"
  Selector/1 -> Selector1/1, Selector3/1, Selector2/1
  Selector2/1 -> Fcn2/1
  Selector3/1 -> normalizza/1(In1)
  Fcn2/1 -> Divide/2
  Abs/1 -> Divide/1
  Selector1/1 -> v_véhic (km/h)5/1, Abs/1
  Look-Up Table/1 -> Mux2/3  "lambda"
  Divide/1 -> Look-Up Table/1
  [Raggio_eff] -> Mux2/2
  Gain1/1 -> Mux2/1
  [Vx1] -> Mux2/4
  Mux2/1 -> Fcn5/1
  Fcn5/1 -> Divide1/1

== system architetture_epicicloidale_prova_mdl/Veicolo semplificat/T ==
  V : Inport
  Bus Creator : BusCreator  Inputs=2
  MATLAB Fcn : MATLABFcn  MATLABFcn=matrice_T  Output1D=off
  Product : Product  Inputs=**  Multiplication=Matrix(*)
  Selector : Selector  Elements=[1 2 3]  InputPortWidth=6
  Selector1 : Selector  Elements=[4 5 6]  InputPortWidth=6
  Xdot : Outport
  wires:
  Bus Creator/1 -> Xdot/1
  Selector/1 -> Bus Creator/1  "Xdot1"
  Selector1/1 -> Bus Creator/2  "Xdot2"
  Product/1 -> Selector1/1, Selector/1
  MATLAB Fcn/1 -> [matT], Product/1
  V/1 -> Product/2
  [thetaM] -> MATLAB Fcn/1

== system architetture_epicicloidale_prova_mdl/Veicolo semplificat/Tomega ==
  V : Inport
  Constant5 : Constant  Value=T_omega
  Product : Product  Inputs=**  Multiplication=Matrix(*)
  Vt : Outport
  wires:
  Product/1 -> Vt/1
  V/1 -> Product/2
  Constant5/1 -> Product/1

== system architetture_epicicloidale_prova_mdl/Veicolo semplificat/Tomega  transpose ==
  T : Inport
  Constant5 : Constant  Value=T_omega
  Product : Product  Inputs=**  Multiplication=Matrix(*)
  Transpose : dspmtrx3/Transpose  Hermitian=off  overflowFlag=on
  Tt : Outport
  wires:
  Transpose/1 -> Product/1
  Constant5/1 -> Transpose/1
  T/1 -> Product/2
  Product/1 -> Tt/1

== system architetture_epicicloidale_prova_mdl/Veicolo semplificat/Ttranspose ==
  F : Inport
  Product : Product  Inputs=**  Multiplication=Matrix(*)
  Transpose : dspmtrx3/Transpose  Hermitian=off  overflowFlag=on
  Ft : Outport
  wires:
  Transpose/1 -> Product/1
  [matT] -> Transpose/1
  F/1 -> Product/2
  Product/1 -> Ft/1

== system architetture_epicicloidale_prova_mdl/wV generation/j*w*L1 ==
  In1 : Inport
  In2 : Inport  Port=2
  Gain1 : Gain  Gain=Kr  Multiplication=Matrix(K*u) (u vector)
  Gain2 : Gain  Gain=Jr  Multiplication=Matrix(K*u) (u vector)
  Gain4 : Gain  Gain=MLb  Multiplication=Matrix(K*u) (u vector)
  Product : Product
  Out1 : Outport
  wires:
  In1/1 -> Gain4/1
  In2/1 -> Gain1/1
  Gain1/1 -> Product/1
  Gain4/1 -> Product/2
  Product/1 -> Gain2/1
  Gain2/1 -> Out1/1

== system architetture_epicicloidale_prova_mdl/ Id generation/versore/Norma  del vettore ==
  In1 : Inport
  Dot Product : simulink/Math Operations/Dot Product  InputSameDT=on  OutDataType=sfix(16)  OutScaling=2^-10  DoSatur=off
  Math Function : Math  Operator=sqrt
  Out1 : Outport
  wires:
  Math Function/1 -> Out1/1
  Dot Product/1 -> Math Function/1
  In1/1 -> Dot Product/2, Dot Product/1

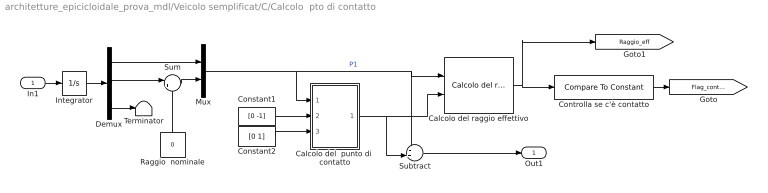
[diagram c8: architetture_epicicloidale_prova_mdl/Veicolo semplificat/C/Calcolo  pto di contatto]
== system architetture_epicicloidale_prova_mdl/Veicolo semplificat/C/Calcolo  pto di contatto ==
  In1 : Inport
  Calcolo del  punto di  contatto : Subsystem  AncestorBlock=|
      | Tire_Soil/Tire-soil contact
      | ENERGETIC/Calcolo versori
      | e punto di contatto C/Subsystem2/Calcolo del 
      | punto di 
      | contatto
  Calcolo del raggio effettivo : Tire_Soil/Tire-soil contact ENERGETIC/Calcolo versori e punto di contatto C/Subsystem2/Calcolo del raggio effettivo
  Constant1 : Constant  Value=[0 -1]
  Constant2 : Constant  Value=[0 1]
  Controlla se c'è contatto : simulink/Logic and Bit Operations/Compare To Constant  relop=<  const=Raggio_Ruota_Ant  LogicOutDataTypeMode=boolean  ZeroCross=off
  Demux : Demux  Outputs=3
  Integrator : Integrator  InitialCondition=[0 Raggio_Ruota_Pos 0]
  Mux : Mux  Inputs=2
  Raggio  nominale : Constant  Orientation=up  Value=0
  Subtract : Sum  Inputs=-+|  OutScaling=2^-10
  Sum : Sum  Inputs=|++
  Terminator : Terminator
  Out1 : Outport
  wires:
  Controlla se c'è contatto/1 -> [Flag_contatto]
  In1/1 -> Integrator/1
  Calcolo del raggio effettivo/1 -> [Raggio_eff], Controlla se c'è contatto/1
  Mux/1 -> Calcolo del  punto di  contatto/1(P1), Calcolo del raggio effettivo/1, Subtract/1  "P1"
  Constant1/1 -> Calcolo del  punto di  contatto/2(r)
  Calcolo del  punto di  contatto/1(Pc) -> Subtract/2, Calcolo del raggio effettivo/2
  Subtract/1 -> Out1/1
  Constant2/1 -> Calcolo del  punto di  contatto/3(n)
  Integrator/1 -> Demux/1
  Sum/1 -> Mux/2
  Demux/1 -> Mux/1
  Raggio  nominale/1 -> Sum/2
  Demux/2 -> Sum/1
  Demux/3 -> Terminator/1

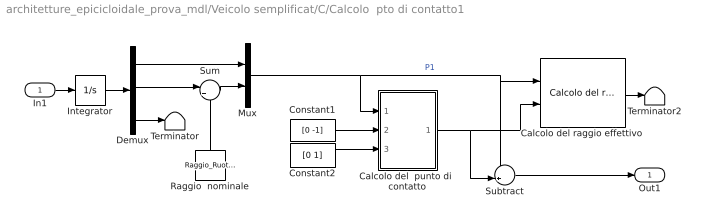
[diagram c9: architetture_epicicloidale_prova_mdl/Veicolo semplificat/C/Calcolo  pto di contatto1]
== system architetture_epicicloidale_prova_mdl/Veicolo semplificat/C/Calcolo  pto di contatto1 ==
  In1 : Inport
  Calcolo del  punto di  contatto : Subsystem  AncestorBlock=|
      | Tire_Soil/Tire-soil contact
      | ENERGETIC/Calcolo versori
      | e punto di contatto C/Subsystem2/Calcolo del 
      | punto di 
      | contatto
  Calcolo del raggio effettivo : Tire_Soil/Tire-soil contact ENERGETIC/Calcolo versori e punto di contatto C/Subsystem2/Calcolo del raggio effettivo
  Constant1 : Constant  Value=[0 -1]
  Constant2 : Constant  Value=[0 1]
  Demux : Demux  Outputs=3
  Integrator : Integrator
  Mux : Mux  Inputs=2
  Raggio  nominale : Constant  Orientation=up  Value=Raggio_Ruota_Pos
  Subtract : Sum  Inputs=-+|  OutScaling=2^-10
  Sum : Sum  Inputs=|++
  Terminator : Terminator
  Terminator2 : Terminator
  Out1 : Outport
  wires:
  In1/1 -> Integrator/1
  Calcolo del raggio effettivo/1 -> Terminator2/1
  Mux/1 -> Calcolo del  punto di  contatto/1(P1), Calcolo del raggio effettivo/1, Subtract/1  "P1"
  Constant1/1 -> Calcolo del  punto di  contatto/2(r)
  Calcolo del  punto di  contatto/1(Pc) -> Calcolo del raggio effettivo/2, Subtract/2
  Subtract/1 -> Out1/1
  Constant2/1 -> Calcolo del  punto di  contatto/3(n)
  Integrator/1 -> Demux/1
  Sum/1 -> Mux/2
  Demux/1 -> Mux/1
  Raggio  nominale/1 -> Sum/2
  Demux/2 -> Sum/1
  Demux/3 -> Terminator/1

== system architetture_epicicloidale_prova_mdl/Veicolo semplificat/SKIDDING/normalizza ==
  In1 : Inport
  Constant : Constant  Value=eps
  Divide : Product  Inputs=*/  OutScaling=2^-10
  Norma  del vettore : Subsystem
  Sum1 : Sum  Inputs=|++
  Out1 : Outport
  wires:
  In1/1 -> Divide/1, Norma  del vettore/1(In1)
  Norma  del vettore/1(Out1) -> Sum1/1
  Sum1/1 -> Divide/2
  Constant/1 -> Sum1/2
  Divide/1 -> Out1/1  "versore"

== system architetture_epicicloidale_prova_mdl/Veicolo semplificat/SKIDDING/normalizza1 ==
  In1 : Inport
  Constant : Constant  Value=eps
  Divide : Product  Inputs=*/  OutScaling=2^-10
  Norma  del vettore : Subsystem
  Sum1 : Sum  Inputs=|++
  Out1 : Outport
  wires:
  In1/1 -> Divide/1, Norma  del vettore/1(In1)
  Norma  del vettore/1(Out1) -> Sum1/1
  Sum1/1 -> Divide/2
  Constant/1 -> Sum1/2
  Divide/1 -> Out1/1  "versore"

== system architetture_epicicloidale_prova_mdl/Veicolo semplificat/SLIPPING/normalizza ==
  In1 : Inport
  Constant : Constant  Value=eps
  Divide : Product  Inputs=*/  OutScaling=2^-10
  Norma  del vettore : Subsystem
  Sum1 : Sum  Inputs=|++
  Out1 : Outport
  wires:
  In1/1 -> Divide/1, Norma  del vettore/1(In1)
  Norma  del vettore/1(Out1) -> Sum1/1
  Sum1/1 -> Divide/2
  Constant/1 -> Sum1/2
  Divide/1 -> Out1/1  "versore"

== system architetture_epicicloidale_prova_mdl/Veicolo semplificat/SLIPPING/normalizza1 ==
  In1 : Inport
  Constant : Constant  Value=eps
  Divide : Product  Inputs=*/  OutScaling=2^-10
  Norma  del vettore : Subsystem
  Sum1 : Sum  Inputs=|++
  Out1 : Outport
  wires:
  In1/1 -> Divide/1, Norma  del vettore/1(In1)
  Norma  del vettore/1(Out1) -> Sum1/1
  Sum1/1 -> Divide/2
  Constant/1 -> Sum1/2
  Divide/1 -> Out1/1  "versore"

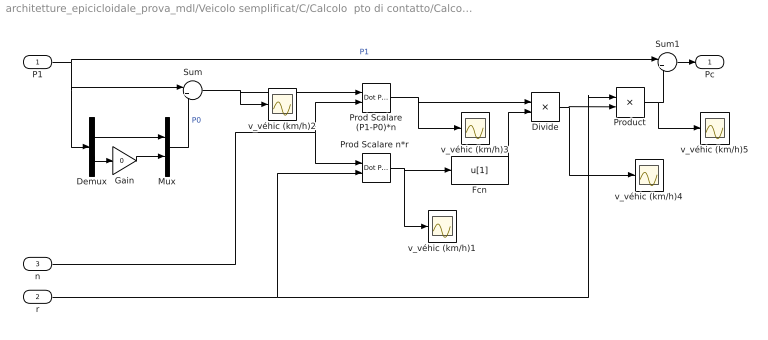
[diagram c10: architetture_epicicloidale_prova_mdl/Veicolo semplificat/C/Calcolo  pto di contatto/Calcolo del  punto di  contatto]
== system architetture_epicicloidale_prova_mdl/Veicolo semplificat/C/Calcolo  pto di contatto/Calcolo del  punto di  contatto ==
  P1 : Inport
  r : Inport  Port=2
  n : Inport  Port=3
  Demux : Demux  Outputs=2
  Divide : Product  Inputs=*/  OutScaling=2^-10
  Fcn : Fcn  Expr=u[1]
  Gain : Gain  Gain=0
  Mux : Mux  Inputs=2
  Prod Scalare (P1-P0)*n : simulink/Math Operations/Dot Product  InputSameDT=on  OutDataType=sfix(16)  OutScaling=2^-10  DoSatur=off
  "Prod Scalare n*r " : simulink/Math Operations/Dot Product  InputSameDT=on  OutDataType=sfix(16)  OutScaling=2^-10  DoSatur=off
  Product : Product
  Sum : Sum  Inputs=|+-
  Sum1 : Sum  Inputs=|+-
  v_véhic (km/h){1..5} (5 alike) : Scope
  Pc : Outport
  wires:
  Gain/1 -> Mux/2
  Mux/1 -> Sum/2  "P0"
  Demux/1 -> Mux/1
  Demux/2 -> Gain/1
  P1/1 -> Demux/1, Sum/1, Sum1/1  "P1"
  r/1 -> "Prod Scalare n*r "/2, Product/1
  Prod Scalare (P1-P0)*n/1 -> v_véhic (km/h)3/1, Divide/1
  "Prod Scalare n*r "/1 -> v_véhic (km/h)1/1, Fcn/1
  Divide/1 -> v_véhic (km/h)4/1, Product/2
  Product/1 -> v_véhic (km/h)5/1, Sum1/2
  Sum1/1 -> Pc/1
  Sum/1 -> v_véhic (km/h)2/1, Prod Scalare (P1-P0)*n/1
  Fcn/1 -> Divide/2
  n/1 -> "Prod Scalare n*r "/1, Prod Scalare (P1-P0)*n/2

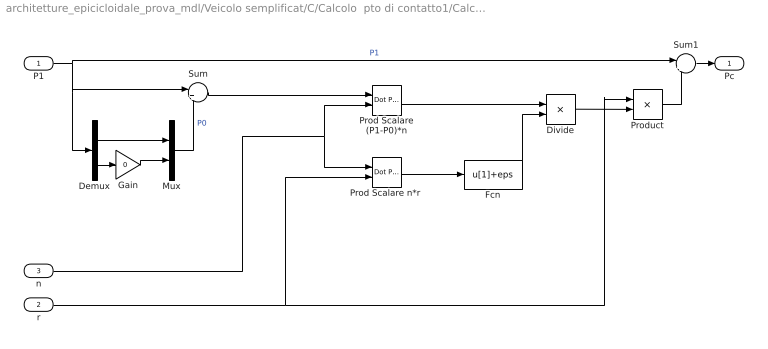
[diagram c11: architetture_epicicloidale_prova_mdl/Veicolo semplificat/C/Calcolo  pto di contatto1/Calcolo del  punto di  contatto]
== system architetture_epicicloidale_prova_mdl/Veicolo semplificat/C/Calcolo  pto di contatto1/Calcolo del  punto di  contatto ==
  P1 : Inport
  r : Inport  Port=2
  n : Inport  Port=3
  Demux : Demux  Outputs=2
  Divide : Product  Inputs=*/  OutScaling=2^-10
  Fcn : Fcn  Expr=u[1]+eps
  Gain : Gain  Gain=0
  Mux : Mux  Inputs=2
  Prod Scalare (P1-P0)*n : simulink/Math Operations/Dot Product  InputSameDT=on  OutDataType=sfix(16)  OutScaling=2^-10  DoSatur=off
  "Prod Scalare n*r " : simulink/Math Operations/Dot Product  InputSameDT=on  OutDataType=sfix(16)  OutScaling=2^-10  DoSatur=off
  Product : Product
  Sum : Sum  Inputs=|+-
  Sum1 : Sum  Inputs=|+-
  Pc : Outport
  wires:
  Gain/1 -> Mux/2
  Mux/1 -> Sum/2  "P0"
  Demux/1 -> Mux/1
  Demux/2 -> Gain/1
  P1/1 -> Demux/1, Sum/1, Sum1/1  "P1"
  r/1 -> "Prod Scalare n*r "/2, Product/1
  Prod Scalare (P1-P0)*n/1 -> Divide/1
  "Prod Scalare n*r "/1 -> Fcn/1
  Divide/1 -> Product/2
  Product/1 -> Sum1/2
  Sum1/1 -> Pc/1
  Sum/1 -> Prod Scalare (P1-P0)*n/1
  Fcn/1 -> Divide/2
  n/1 -> "Prod Scalare n*r "/1, Prod Scalare (P1-P0)*n/2

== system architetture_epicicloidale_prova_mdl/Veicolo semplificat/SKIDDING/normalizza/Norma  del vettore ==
  In1 : Inport
  Dot Product : simulink/Math Operations/Dot Product  InputSameDT=on  OutDataType=sfix(16)  OutScaling=2^-10  DoSatur=off
  Math Function : Math  Operator=sqrt
  Out1 : Outport
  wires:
  In1/1 -> Dot Product/1, Dot Product/2
  Dot Product/1 -> Math Function/1
  Math Function/1 -> Out1/1

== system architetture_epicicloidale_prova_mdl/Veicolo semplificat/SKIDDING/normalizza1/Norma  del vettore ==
  In1 : Inport
  Dot Product : simulink/Math Operations/Dot Product  InputSameDT=on  OutDataType=sfix(16)  OutScaling=2^-10  DoSatur=off
  Math Function : Math  Operator=sqrt
  Out1 : Outport
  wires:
  In1/1 -> Dot Product/1, Dot Product/2
  Dot Product/1 -> Math Function/1
  Math Function/1 -> Out1/1

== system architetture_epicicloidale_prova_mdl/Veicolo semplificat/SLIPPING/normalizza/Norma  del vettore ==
  In1 : Inport
  Dot Product : simulink/Math Operations/Dot Product  InputSameDT=on  OutDataType=sfix(16)  OutScaling=2^-10  DoSatur=off
  Math Function : Math  Operator=sqrt
  Out1 : Outport
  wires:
  In1/1 -> Dot Product/1, Dot Product/2
  Dot Product/1 -> Math Function/1
  Math Function/1 -> Out1/1

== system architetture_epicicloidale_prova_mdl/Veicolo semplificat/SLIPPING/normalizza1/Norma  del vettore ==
  In1 : Inport
  Dot Product : simulink/Math Operations/Dot Product  InputSameDT=on  OutDataType=sfix(16)  OutScaling=2^-10  DoSatur=off
  Math Function : Math  Operator=sqrt
  Out1 : Outport
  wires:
  In1/1 -> Dot Product/1, Dot Product/2
  Dot Product/1 -> Math Function/1
  Math Function/1 -> Out1/1
